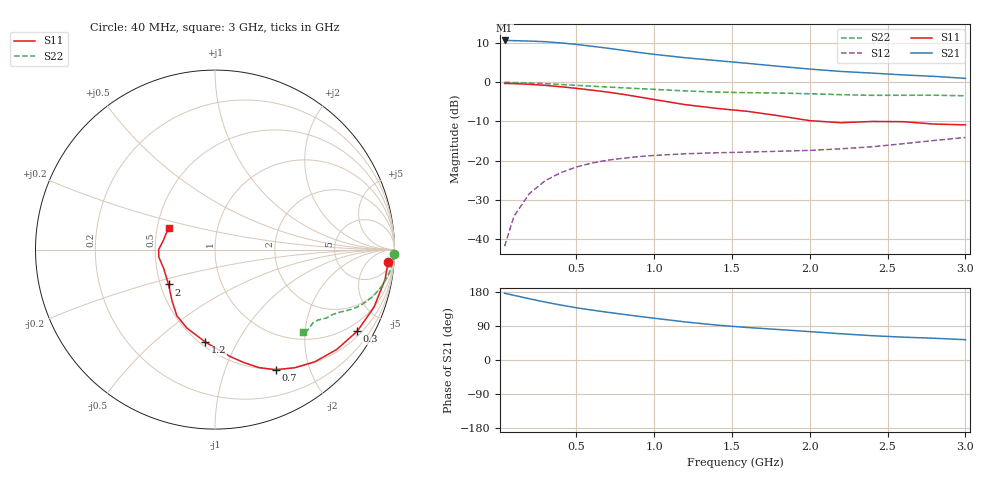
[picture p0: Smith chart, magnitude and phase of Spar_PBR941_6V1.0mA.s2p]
! Filename:  PBR941K.S2P  Version:  3.0
! NXP part #:  PBR941  Date: July 1998
! Bias condition:  Vce=6V, Ic=1.0mA
#  MHz  S  MA  R 50
! Freq  S11  S21  S12  S22
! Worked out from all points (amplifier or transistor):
!   21 points, 40 MHz to 3 GHz, reference 50 ohm
!   highest |S21| = 10.7 dB at 40 MHz (marker M1)
!   |S21| within 3 dB of that: start of sweep to 890.9 MHz
!   unconditionally stable (mu >= 1): 1.914 GHz to end of sweep
!   at 300 MHz: K = 0.18, MSG = 17.8 dB, |S12| = -25.2 dB
!   at 1 GHz: K = 0.54, MSG = 12.9 dB, |S12| = -18.7 dB
!   at 3 GHz: K = 1.07, MAG = 5.9 dB, |S12| = -14.1 dB
!   lowest NFmin = 0.99 dB at 500 MHz
!   S11 on the Smith chart (normalised r, x): 40 MHz: 11, -23; 300 MHz: 0.66, -3.64; 700 MHz: 0.49, -1.51; 1.2 GHz: 0.53, -0.75; 2 GHz: 0.55, -0.24; 3 GHz: 0.57, +0.15
40  0.967 -4.0  3.419 176.2  0.008079 87.1  0.9973 -1.5
100  0.9619 -10.0  3.399 170.6  0.01942 83.9  0.9935 -3.8
200  0.9421 -19.9  3.358 161.5  0.03807 77.8  0.9801 -7.5
300  0.9137 -29.9  3.296 152.9  0.05522 72.9  0.9609 -11.0
400  0.8774 -39.4  3.182 145.1  0.07008 68.4  0.9383 -14.1
500  0.8367 -48.3  3.046 137.9  0.08264 64.3  0.9145 -16.8
600  0.794 -56.0  2.885 131.8  0.09304 61.2  0.8912 -19.0
700  0.7503 -63.1  2.727 126.1  0.1012 58.6  0.8704 -20.8
800  0.7022 -69.5  2.563 120.6  0.1071 56.3  0.8505 -22.3
900  0.6506 -75.5  2.407 115.3  0.1124 54.5  0.8307 -23.5
1000  0.6023 -81.8  2.274 110.3  0.1163 53.3  0.8121 -24.7
1200  0.5181 -95.9  2.057 100.5  0.1222 51.6  0.7761 -26.7
1400  0.4647 -109.6  1.894 92.2  0.1258 51.0  0.7498 -28.8
1600  0.4253 -120.0  1.745 85.7  0.1285 53.2  0.7364 -30.4
1800  0.374 -129.7  1.6 80.4  0.1316 56.3  0.7288 -31.6
2000  0.3236 -143.1  1.474 74.9  0.135 59.8  0.7138 -32.7
2200  0.3046 -160.1  1.375 69.3  0.1415 63.4  0.6944 -34.4
2400  0.3159 -172.5  1.31 64.1  0.15 67.5  0.6816 -36.9
2600  0.3139 180.0  1.242 60.3  0.1642 72.0  0.682 -39.5
2800  0.2926 170.2  1.19 57.3  0.1806 75.5  0.6835 -41.4
3000  0.2861 154.7  1.121 53.6  0.1973 77.8  0.6715 -42.8
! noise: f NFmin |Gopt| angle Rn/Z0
500  0.992  0.723  19.23  0.499
900  1.034  0.605  30.41  0.468
1000  1.23  0.523  36.2  0.51
2000  2.13  0.341  105.5  0.253
